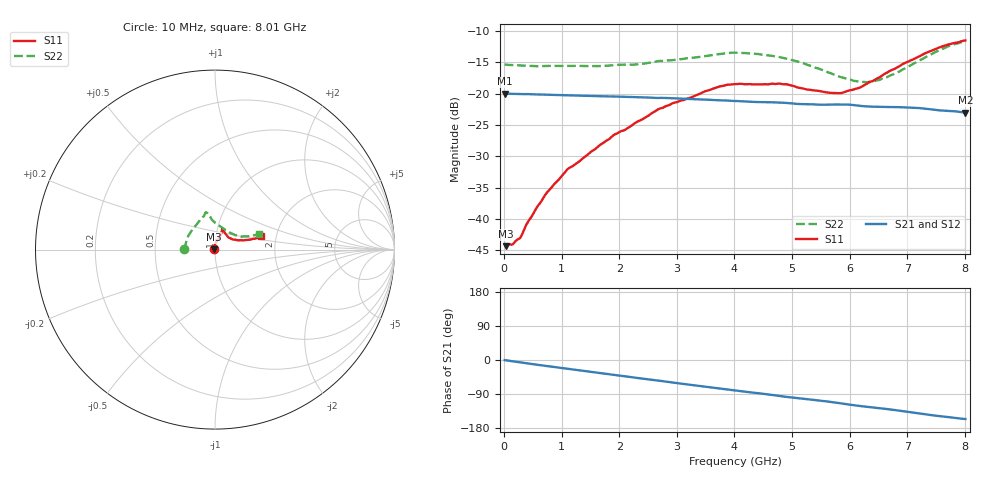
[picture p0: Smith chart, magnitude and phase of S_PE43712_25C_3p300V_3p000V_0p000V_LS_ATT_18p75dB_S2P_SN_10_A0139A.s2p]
! DEVICE ID: PE43712
! File Path: z:\PE43713\PE43713_CHAR_NOM_04292014\AMB\3p300\LS_ATT_18p75dB\PE43713_AMB_3p300V_3p000V_0p000V_LS_ATT_18p75dB_S2P_SN_10_A0139A.s2p
! Serial: 10
! Lot: A0139A
! Temp: 25C
! VDD: 3.300
! VSS: 0.000
! Control_Hi: 3.000
! Control_Lo: 0.000
! Attenuation Step: 18.75dB
! Port 1: RF1
! Port 2: RF2
! ThroughPath:1-2
! IDD: 0.0001464982
! ISS: -1.794e-007
#  Hz  S  RI  R  50
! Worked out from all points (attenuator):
!   801 points, 10 MHz to 8.01 GHz, reference 50 ohm
!   highest |S21| = -19.98 dB at 10 MHz (marker M1); lowest = -23.0 dB at 8.01 GHz (marker M2)
!   lowest |S11| = -44.3 dB at 30 MHz (marker M3), VSWR 1.01, Z = 49.4 + j0.136 ohm
!   |S11| at or under -10 dB: start of sweep to end of sweep
!   |S22| runs from -18.2 to -11.7 dB; largest |S21 - S12| = 0.00039
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1e7  -0.00627 0.000562  0.1002 -0.000532  0.1002 -0.000496  -0.1712 0.00121
3e7  -0.00591 0.00137  0.1002 -0.00127  0.1002 -0.00128  -0.1706 0.003
1.5e8  -0.00506 0.00372  0.0998 -0.00595  0.0998 -0.00594  -0.169 0.0113
2.7e8  -0.00435 0.00547  0.0991 -0.0105  0.0991 -0.0105  -0.1674 0.0181
4.2e8  -0.00402 0.00867  0.0981 -0.0161  0.098 -0.0161  -0.1654 0.0268
7.4e8  -0.00371 0.0157  0.0945 -0.0271  0.0945 -0.0271  -0.1602 0.0471
1.1e9  -0.00231 0.0248  0.0891 -0.0384  0.0892 -0.0384  -0.1521 0.0687
1.35e9  0.000106 0.03  0.085 -0.0456  0.085 -0.0456  -0.1453 0.0818
1.91e9  0.00879 0.0462  0.0736 -0.0602  0.0736 -0.0601  -0.1243 0.1152
2.34e9  0.018 0.0577  0.063 -0.0697  0.063 -0.0697  -0.1046 0.1366
2.68e9  0.0268 0.0705  0.0539 -0.0753  0.0539 -0.0753  -0.0877 0.16
3.71e9  0.0389 0.1061  0.0235 -0.0856  0.0235 -0.0856  -0.0555 0.1989
4.01e9  0.0401 0.1125  0.0147 -0.0864  0.0147 -0.0864  -0.0525 0.2064
4.79e9  0.0437 0.1123  -0.0073 -0.0846  -0.00734 -0.0847  -0.0341 0.1928
5.35e9  0.0562 0.0909  -0.0215 -0.0796  -0.0214 -0.0795  -0.0158 0.1648
5.87e9  0.0769 0.0665  -0.0342 -0.0744  -0.0342 -0.0744  0.0233 0.1331
6.29e9  0.1058 0.0554  -0.0434 -0.0664  -0.0433 -0.0664  0.0675 0.1035
6.41e9  0.1146 0.0542  -0.0453 -0.0645  -0.0452 -0.0645  0.0807 0.0951
6.68e9  0.1414 0.052  -0.0504 -0.0599  -0.0503 -0.06  0.1122 0.0807
7.55e9  0.2252 0.0622  -0.0625 -0.0391  -0.0625 -0.0392  0.2079 0.078
7.81e9  0.2441 0.0698  -0.0643 -0.0336  -0.0642 -0.0336  0.2334 0.0842
8.01e9  0.2554 0.0761  -0.0645 -0.0291  -0.0644 -0.0292  0.2451 0.0854
